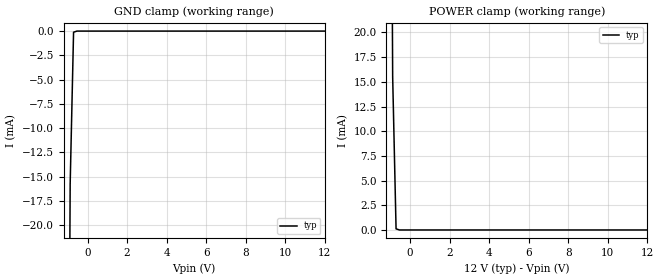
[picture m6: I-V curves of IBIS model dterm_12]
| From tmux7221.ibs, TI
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| dterm_12
[Model]   dterm_12
Model_type   Terminator
|   typ   min   max
C_comp   1.008417e-11   NA   NA
[Voltage Range]   12   NA   NA
[Temperature Range]   27   NA   NA
[Power Clamp Reference]   12   NA   NA
[GND Clamp Reference]   0   NA   NA
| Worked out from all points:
|   GND clamp passes 1 mA (typ) near -0.72 V on its own axis
|   POWER clamp passes 1 mA (typ) near -0.72 V on its own axis
[GND Clamp]
|   Voltage   I(typ)   I(min)   I(max)
-5V       -4.78A     NA         NA
-1.051V   -81.7mA    NA         NA
-878.8mV  -15.77mA   NA         NA
-707.1mV  -116.4uA   NA         NA
-535.4mV  -304.8nA   NA         NA
12V       416pA      NA         NA
[POWER Clamp]
|   Voltage   I(typ)   I(min)   I(max)
-5V       5.371A     NA         NA
-1.05V    80.18mA    NA         NA
-878.8mV  15.49mA    NA         NA
-707.1mV  114.6uA    NA         NA
-535.4mV  269nA      NA         NA
12V       -416.3pA   NA         NA
